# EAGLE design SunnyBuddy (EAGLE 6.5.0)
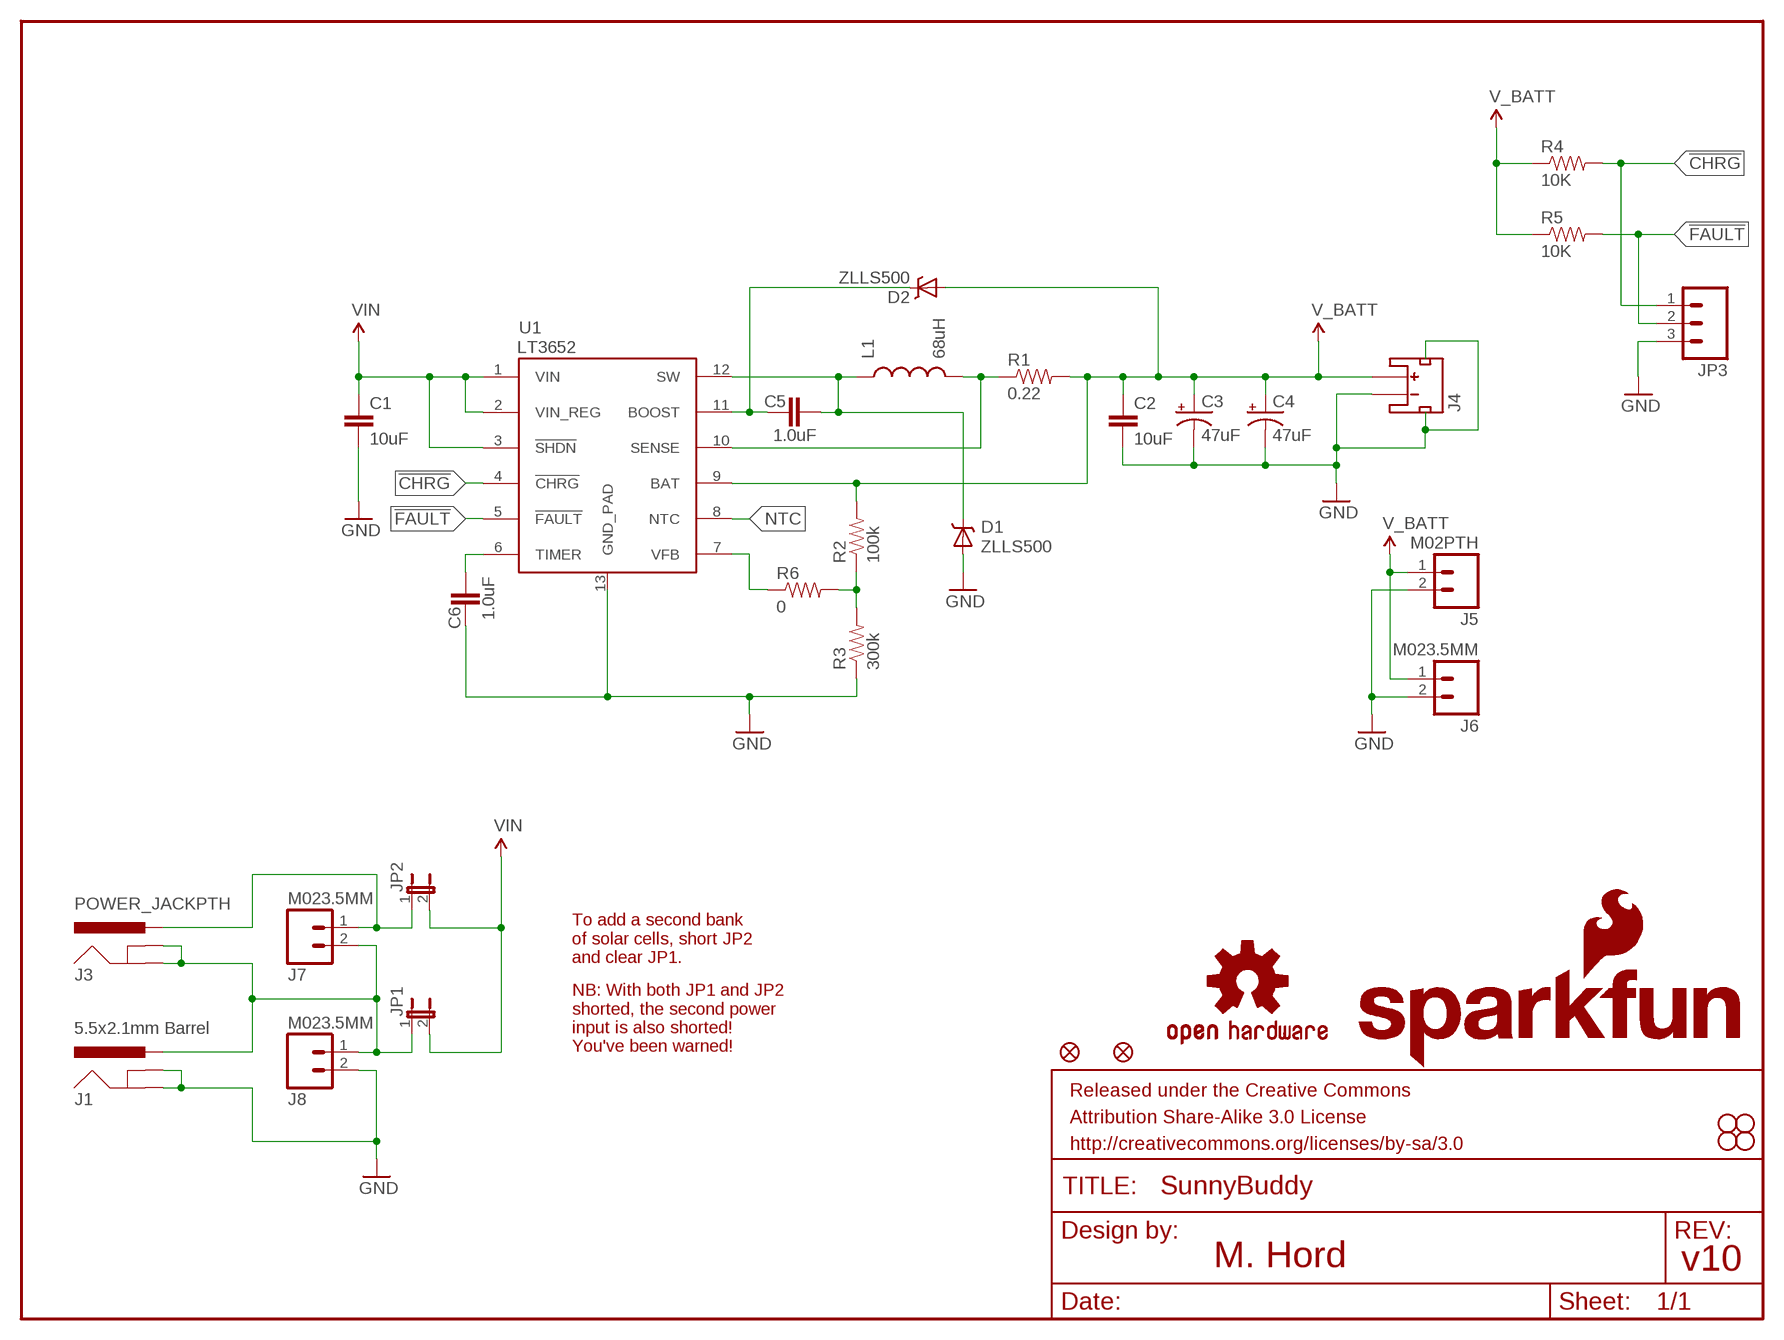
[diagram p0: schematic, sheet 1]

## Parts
C1  10uF  10UF50V20%(1210)  [1210]
C2  10uF  10UF-6.3V-20%(1206)  [1206]
C3  47uF  47UF-TANT  [EIA3528]
C4  47uF  47UF-TANT  [EIA3528]
C5  1.0uF  1.0UF-16V-10%(0603)  [0603-CAP]
C6  1.0uF  1.0UF-16V-10%(0603)  [0603-CAP]
D1  ZLLS500  ZLLS500ZLLS500  [SOT23]
D2  ZLLS500  ZLLS500ZLLS500  [SOT23]
FID1  FIDUCIAL1X2  [FIDUCIAL-1X2]
FID2  FIDUCIAL1X2  [FIDUCIAL-1X2]
FRAME1  FRAME-LETTER  [CREATIVE_COMMONS]
J1  5.5x2.1mm Barrel  POWER_JACKSMD  [POWER_JACK_SMD]
J3  POWER_JACKPTH  [POWER_JACK_PTH]
J4  JST_2MM_MALE  [JST-2-SMD]
J5  M02PTH  [1X02]
J6  M023.5MM  [SCREWTERMINAL-3.5MM-2]
J7  M023.5MM  [SCREWTERMINAL-3.5MM-2]
J8  M023.5MM  [SCREWTERMINAL-3.5MM-2]
JP1  JUMPER-2SMD-NC  [SJ_2S]
JP2  JUMPER-2SMD-NO  [SJ_2S-NO]
JP3  M03PTH  [1X03]
L1  68uH  INDUCTOR68UH-1A  [CR75]
LOGO1  SFE_LOGO_NAME_FLAME.2_INCH  [SFE_LOGO_NAME_FLAME_.2]
LOGO2  OSHW-LOGOM  [OSHW-LOGO-M]
R1  0.22  0.22OHM1/4W1%(0805)  [0805]
R2  100k  100KOHM1/10W1%(0603)  [0603-RES]
R3  300k  300KOHM-1/10W-1%(0603)  [0603-RES]
R4  10K  10KOHM1/10W1%(0603)0603  [0603-RES]
R5  10K  10KOHM1/10W1%(0603)0603  [0603-RES]
R6  0  0OHM1/10W5%(0603)  [0603]
STANDOFF1  STAND-OFF  [STAND-OFF]
STANDOFF2  STAND-OFF  [STAND-OFF]
STANDOFF3  STAND-OFF  [STAND-OFF]
STANDOFF4  STAND-OFF  [STAND-OFF]
U1  LT3652  [MSOP-12_GND]

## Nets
!CHRG: JP3.1 R4.2 U1.4(!CHRG)
!FAULT: JP3.2 R5.2 U1.5(!FAULT)
BOOST: C5.1 D2.3(C) U1.11(BOOST)
FB: R2.1 R3.2 R6.2
GND: C1.2 C2.2 C3.C(-) C4.C(-) C6.1 D1.1(A) J1.GND(GNDBREAK) J1.P$4(GND) J4.1(-) J4.NC1(PAD1) J4.NC2(PAD2) J5.2 J6.2 J8.2 JP3.3 R3.1 U1.13(GND_PAD)
N$3: R6.1 U1.7(VFB)
N$8: J1.VIN0(PWR) J3.GND J3.GNDBREAK J7.2 J8.1 JP1.1
NTC: U1.8(NTC)
SENSE: L1.P$2 R1.1 U1.10(SENSE)
SFSASDF: J3.PWR J7.1 JP2.1
SW: C5.2 D1.3(C) L1.P$1 U1.12(SW)
TIMER: C6.2 U1.6(TIMER)
V_BATT: C2.1 C3.A(+) C4.A(+) D2.1(A) J4.2(+) J5.1 J6.1 R1.2 R2.2 R4.1 R5.1 U1.9(BAT)
VIN: C1.1 JP1.2 JP2.2 U1.1(VIN) U1.2(VIN_REG) U1.3(!SHDN)

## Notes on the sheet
- To add a second bank
  of solar cells, short JP2
  and clear JP1.
- NB: With both JP1 and JP2
  shorted, the second power
  input is also shorted!
  You've been warned!
- M. Hord | v10

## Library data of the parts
C1 = SparkFun-Capacitors:10UF50V20%(1210): CAP-09824; PROD_ID: CAP-09824
C2 = SparkFun-Capacitors:10UF-6.3V-20%(1206): Ceramic; PROD_ID: CAP-10057
C3 C4 = SparkFun-Capacitors:47UF-TANT: 47uF Tantalum SMT; PROD_ID: CAP-08310
C5 C6 = SparkFun-Capacitors:1.0UF-16V-10%(0603): CAP-00868; PROD_ID: CAP-00868
D1 D2 = SparkFun-DiscreteSemi:ZLLS500: 700mA 40V SOT-23 Schottky; PROD_ID: DIO-08411
FID1 FID2 = SparkFun-Aesthetics:FIDUCIAL: Fiducial Alignment Points
FRAME1 = SparkFun-Aesthetics:FRAME-LETTER: Schematic Frame
J1 = SparkFun-Connectors:POWER_JACK: Power Jack This is the standard 5.5mm barrel jack for power. The PTH is the most common, proven, reliable, footprint. The Slot footprint only works if the mill layer is transmitted to the PCB fab house so be warned. Spark Fun Electronics SKU : PRT-00119 SMT: CONN-08106 Mating wall wart : TOL-00298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; PROD_ID: CONN-08106
J3 = SparkFun-Connectors:POWER_JACK: Power Jack This is the standard 5.5mm barrel jack for power. The PTH is the most common, proven, reliable, footprint. The Slot footprint only works if the mill layer is transmitted to the PCB fab house so be warned. Spark Fun Electronics SKU : PRT-00119 SMT: CONN-08106 Mating wall wart : TOL-00298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
J4 = SparkFun-Connectors:JST_2MM_MALE: Mates to single-cell LiPo batteries. CONN-08352; PROD_ID: CONN-08352
J5-J8 = SparkFun-Connectors:M02: Standard 2-pin 0.1" header. Use with
JP1 JP2 = SparkFun-Passives:JUMPER-2: Jumper
JP3 = SparkFun-Connectors:M03: Header 3 Standard 3-pin 0.1" header. Use with straight break away headers (SKU : PRT-00116), right angle break away headers (PRT-00553), swiss pins (PRT-00743), machine pins (PRT-00117), and female headers (PRT-00115). Molex polarized connector foot print use with SKU : PRT-08232 with associated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
L1 = SparkFun-Passives:INDUCTOR: Inductors; PROD_ID: NDUC-09739
LOGO1 = SparkFun-Aesthetics:SFE_LOGO_NAME_FLAME: SFE Logo, name and flame
LOGO2 = SparkFun-Aesthetics:OSHW-LOGO: Open Source Hardware Logo This logo indicates the piece of hardware it is found on incorporates a OSHW license and/or adheres to the definition of open source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
R1 = SparkFun-Resistors:0.22OHM1/4W1%(0805): RES-09883; PROD_ID: RES-09883
R2 = SparkFun-Resistors:100KOHM1/10W1%(0603): RES-07828; PROD_ID: RES-07828
R3 = SparkFun-Resistors:300KOHM-1/10W-1%(0603): RES-10809; PROD_ID: RES-10809
R4 R5 = SparkFun-Resistors:10KOHM1/10W1%(0603): RES-00824; PROD_ID: RES-00824
R6 = SparkFun-Resistors:0OHM1/10W5%(0603): RES-08609; PROD_ID: RES-08609
STANDOFF1-STANDOFF4 = SparkFun-Electromechanical:STAND-OFF: #4 Stand Off
U1 = SparkFun-PowerIC:LT3652: LT3652 MPPT Solar Charge Controller 5V-32V smart charger for batteries up to 14.4V

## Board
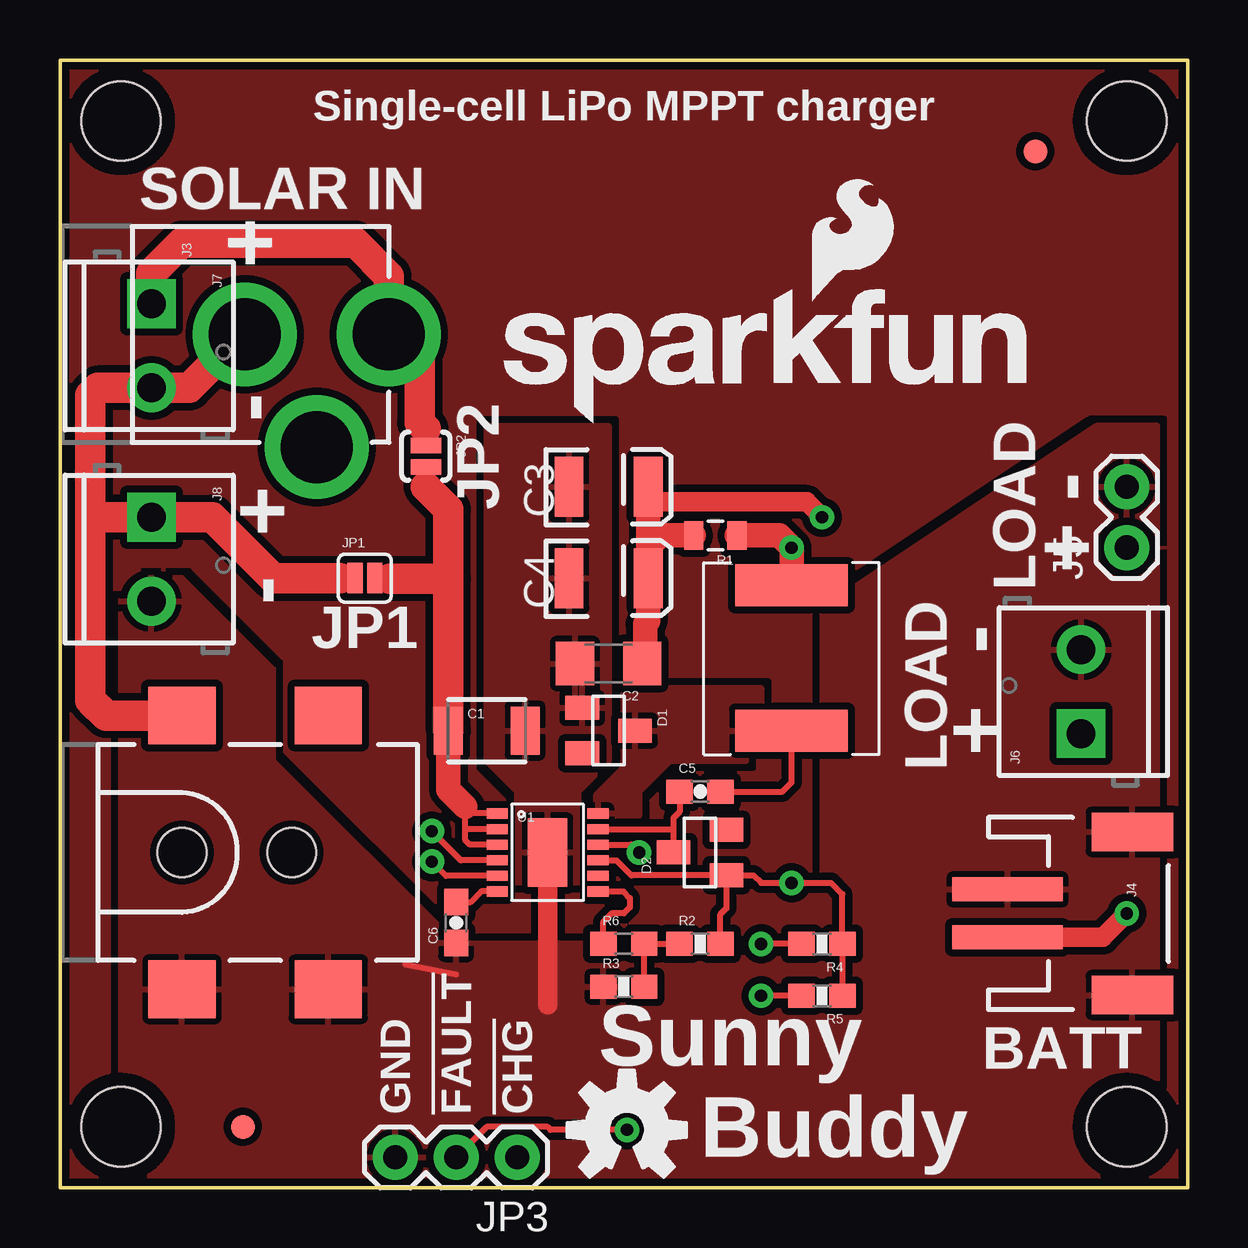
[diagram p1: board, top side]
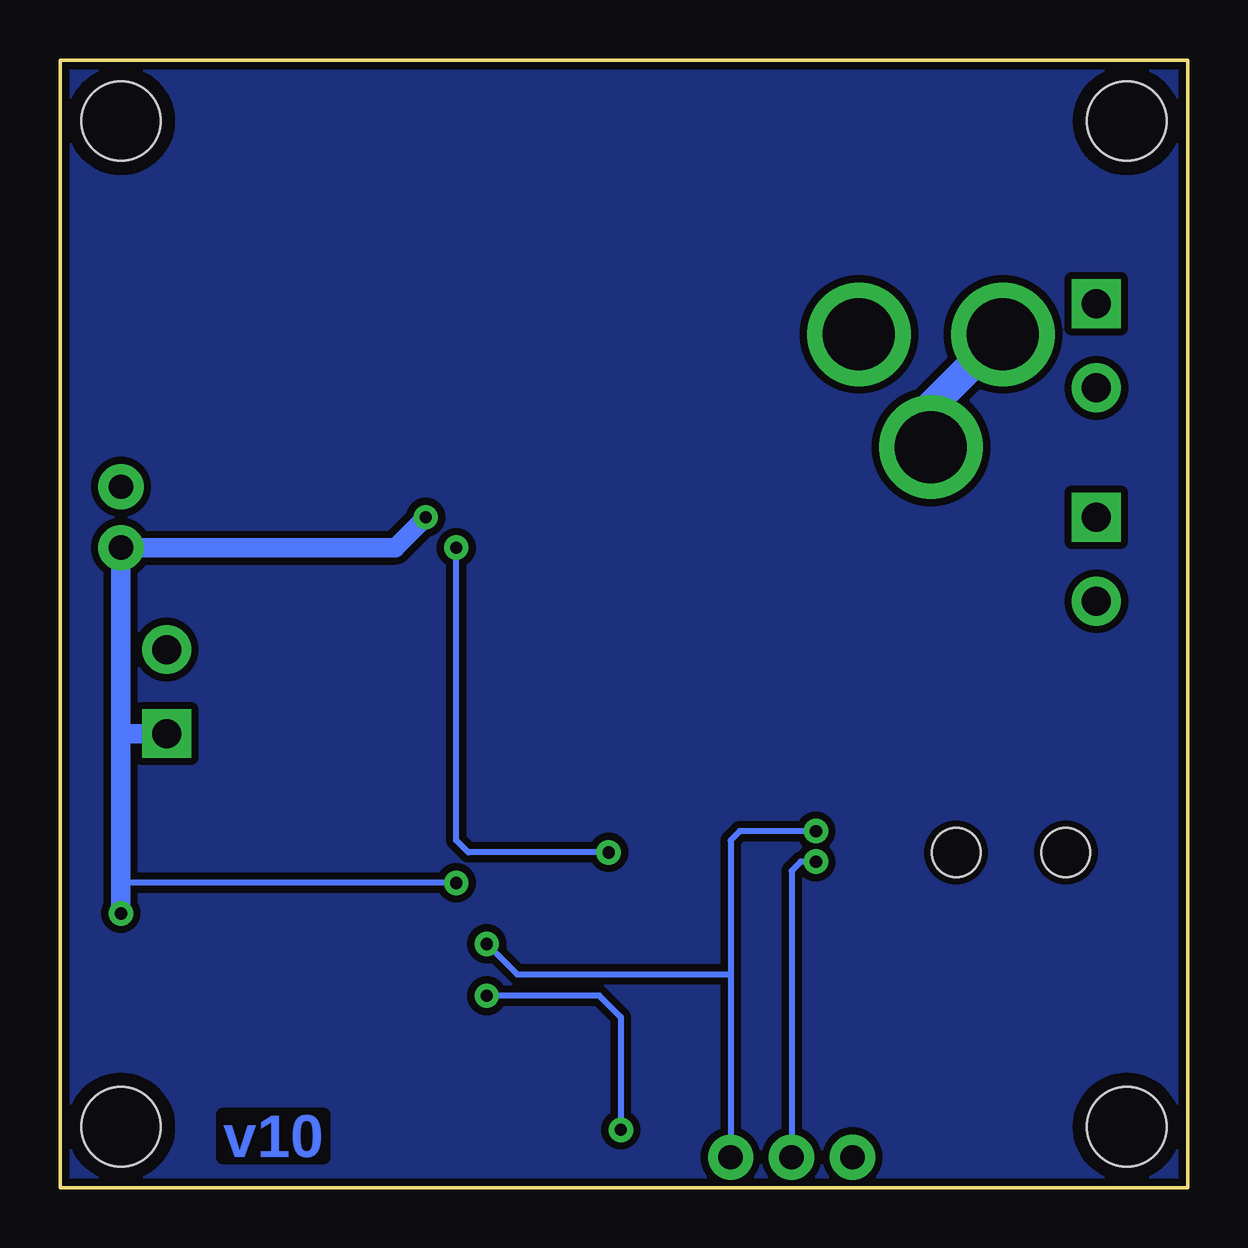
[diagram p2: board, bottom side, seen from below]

Size 46.99 x 46.99 mm. Coordinates in mm from the lower left corner, seen from the top.
Outline: 0,46.99 46.99,46.99 46.99,0 0,0 0,46.99
Copper layers (1*16): Top 0.035mm / dielectric 1.5mm / Bottom 0.035mm
Design rules "Sparkfun": minimum track width 8mil, minimum drill 20mil, track to track 8mil, track to pad 8mil, pad to pad 8mil, via to via 8mil, smd to smd 8mil, copper to edge 8mil, drill to drill 8mil, minimum pad ring 12mil, minimum via ring 10mil, stop-mask expansion 4mil, vias tented up to drill 20mil, thermal gap 10mil

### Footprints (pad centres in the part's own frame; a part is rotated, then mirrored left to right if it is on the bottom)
1210 = smd 1.2 x 2: 1 -1.6,0; 2 1.6,0
1206 = smd 1.6 x 1.8: 1 -1.4,0; 2 1.4,0
EIA3528 = smd 1.2 x 2.5: A 1.65,0; C -1.65,0
0603-CAP = smd 1.1 x 1: 1 -0.85,0; 2 0.85,0
SOT23 = smd 1 x 1.4: 1 -0.95,-1.1; 2 0.95,-1.1; 3 0,1.1
FIDUCIAL-1X2 = smd 1 x 1: 1 0,0
POWER_JACK_SMD = smd 2.8 x 2.4: GND 0,-5.7; P$4 6.1,-5.7; VIN0 0,5.7; VIN1 6.1,5.7 | hole 2.032: 0,0; 4.572,0
POWER_JACK_PTH = drill 2.997 pad 4.318: GND 0,7.7; GNDBREAK 4.7,10.7; PWR 0,13.7
JST-2-SMD = smd 1 x 4.6: 1 -1,-3.7; 2 1,-3.7 | smd 1.6 x 3.4: NC1 -3.4,1.5; NC2 3.4,1.5
1X02 = drill 1.016 pad 1.88: 1 0,0; 2 2.54,0
SCREWTERMINAL-3.5MM-2 = drill 1.2 pad 2.032 square: 1 0,0 | drill 1.2 pad 2.032: 2 3.5,0
SJ_2S = smd 0.635 x 1.27: 1 -0.412,0; 2 0.412,0
SJ_2S-NO = smd 0.635 x 1.27: 1 -0.45,0; 2 0.45,0
1X03 = drill 1.016 pad 1.88: 1 0,0; 2 2.54,0; 3 5.08,0
CR75 = smd 1.75 x 4.7: P$1 0,0; P$2 6.05,0
0805 = smd 0.8 x 1.2: 1 -0.9,0; 2 0.9,0
0603-RES = smd 1.1 x 1: 1 -0.85,0; 2 0.85,0
0603 = smd 1.1 x 1: 1 -0.85,0; 2 0.85,0
STAND-OFF = hole 3.302: 0,0
MSOP-12_GND = smd 0.889 x 0.42: 1 -2.1,1.625; 2 -2.1,0.975; 3 -2.1,0.325; 4 -2.1,-0.325; 5 -2.1,-0.975; 6 -2.1,-1.625; 7 2.1,-1.625; 8 2.1,-0.975; 9 2.1,-0.325; 10 2.1,0.325; 11 2.1,0.975; 12 2.1,1.625 | smd 1.651 x 2.845: 13 0,0

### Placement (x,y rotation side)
C1  17.78,19.05 0 top
C2  22.86,21.84 180 top
C3  22.86,29.21 0 top
C4  22.86,25.4 0 top
C5  26.67,16.51 0 top
C6  16.51,11.05 90 top
D1  22.86,19.05 270 top
D2  26.67,13.97 90 top
FID1  7.62,2.54 0 top
FID2  40.64,43.18 0 top
FRAME1  not placed on the board
J1  5.08,13.97 0 top
J3  0,35.56 270 top
J4  43.18,11.43 270 top
J5  44.45,26.67 90 top
J6  42.55,18.92 90 top
J7  3.81,36.83 270 top
J8  3.81,27.94 270 top
JP1  12.7,25.4 0 top
JP2  15.24,30.48 270 top
JP3  19.05,1.27 180 top
L1  30.48,19.05 90 top
LOGO1  17.78,31.75 0 top
LOGO2  23.62,2.41 0 top
R1  27.3,27.18 180 top
R2  26.67,10.16 0 top
R3  23.5,8.38 0 top
R4  31.75,10.16 180 top
R5  31.75,8 180 top
R6  23.5,10.16 0 top
STANDOFF1  2.54,2.54 0 top
STANDOFF2  2.54,44.45 0 top
STANDOFF3  44.45,44.45 0 top
STANDOFF4  44.45,2.54 0 top
U1  20.32,13.97 0 top

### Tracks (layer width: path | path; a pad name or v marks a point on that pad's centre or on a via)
!CHRG  (via drill 0.51)
  Top 0.254: U1.4 16.71,13.64 v15.49,14.86 | R4.2 v29.21,10.16
  Bottom 0.254: v15.49,14.86 18.67,14.86 19.05,14.48 19.05,8.89 | 19.05,8.89 JP3.1 | 19.05,8.89 27.94,8.89 v29.21,10.16
!FAULT  (via drill 0.51)
  Top 0.254: U1.5 16.09,12.99 v15.49,13.59 | v23.62,2.41 20.45,2.41 20.32,2.54 17.78,2.54 JP3.2 | R5.2 v29.21,8
  Bottom 0.254: v15.49,13.59 16.13,13.59 16.51,13.21 JP3.2 | v23.62,2.41 23.62,7.11 24.51,8 v29.21,8
BOOST
  Top 0.254: D2.3 25.57,14.86 | 25.57,14.86 25.57,15.41 25.82,15.66 C5.1 | U1.11 25.48,14.95 25.57,14.86
FB
  Top 0.254: R2.1 R6.2 R3.2
GND
  Top 0.254: 14.39,9.31 16.51,8.89
  Top 0.813: U1.13 20.32,7.62
  pour Top (isolate 0.305): 43.18,31.75 31.75,24.13 31.75,12.7 29.21,10.16 16.51,10.16 8.89,17.78 8.89,21.59 5.08,25.4 2.54,25.4 2.54,0 45.72,0 45.72,31.75
  pour Top (isolate 0.305): 22.86,31.75 22.86,17.78 21.59,16.51 21.59,12.7 19.05,12.7 19.05,16.51 17.78,17.78 17.78,31.75
N$1
  pour Top (isolate 0.305, rank 2, no thermals): 0,46.99 46.99,46.99 46.99,0 0,0
N$2
  pour Bottom (isolate 0.305, rank 2, no thermals): 0,46.99 46.99,46.99 46.99,0 0,0
N$3
  Top 0.254: U1.7 23.47,12.35 23.75,12.06 23.75,11.68 23.5,11.43 22.99,11.43 22.64,11.09 R6.1
N$8
  Top 0.254: J3.GND 7.62,35.56 | 11.68,25.4 JP1.1
  Top 1.27: 7.62,35.56 5.39,33.33 J7.2 1.58,33.33 1.27,33.02 1.27,27.94 | 1.27,27.94 1.27,20.32 1.92,19.67 J1.VIN0 | 11.68,25.4 8.89,25.4 6.35,27.94 J8.1 1.27,27.94
  Bottom 1.27: J3.GNDBREAK 10.7,32.56 J3.GND
SENSE  (via drill 0.51)
  Top 0.254: U1.10 23.8,14.29 v24.13,13.97
  Top 1.016: R1.1 29.97,27.18 v30.48,26.67 L1.P$2
  Bottom 0.254: v24.13,13.97 29.97,13.97 30.48,14.48 v30.48,26.67
SFSASDF
  Top 0.254: JP2.1 15.24,31.62
  Top 1.27: J7.1 3.81,38.1 5.08,39.37 12.32,39.37 13.7,37.99 J3.PWR 14.99,34.42 14.99,31.88 15.24,31.62
SW
  Top 0.254: C5.2 30.1,16.51 30.48,16.89 L1.P$1
  pour Top (isolate 0.305): 23.5,20.83 29.21,20.83 29.21,18.41 28.57,17.78 25.4,17.78 24.13,16.51 24.13,15.49 22.35,15.49 22.35,16.38 23.5,17.53
TIMER
  Top 0.254: U1.6 17.55,12.35 17.11,11.9 C6.2
V_BATT  (via drill 0.51)
  Top 0.254: U1.9 23.18,13.64 23.81,13.02 D2.1 | D2.1 28.89,13.02 29.21,12.7 v30.48,12.7 32.13,12.7 32.6,12.23 R4.1 R5.1 | 24.13,21.97 C2.1 | D2.1 27.77,11.64 27.52,11.39 R2.2
  Top 0.813: J4.2 43.45,10.43 v44.45,11.43 | C3.A 24.51,28.45 24.64,28.57 31.11,28.57 v31.75,27.94
  Top 1.016: 24.51,28.45 24.51,26.67 | 24.51,26.67 C4.A 24.51,23.62 24.38,23.5 24.38,21.97 C2.1 | R1.2 25.02,27.18 24.51,26.67
  Bottom 0.254: v30.48,12.7 44.45,12.7
  Bottom 0.813: v44.45,11.43 44.45,12.7 44.45,19.05 | 44.45,19.05 J5.1 33.02,26.67 v31.75,27.94 | J6.1 44.32,18.92 44.45,19.05
VIN
  Top 0.254: 13.73,25.39 13.72,25.4 JP1.2 | JP2.2 15.24,29.21 | U1.1 17.17,15.6 16.89,15.88 16.89,14.99 | U1.3 17.07,14.29 16.89,14.48 16.89,14.99 | U1.2 16.93,14.95 16.89,14.99
  Top 1.016: C1.1 16.18,16.59 16.89,15.88
  Top 1.27: C1.1 16.18,25.39 | 16.18,25.39 13.73,25.39 | 16.18,25.39 16.18,28.27 15.24,29.21

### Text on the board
Bottom: v10
tPlace: Single-cell LiPo MPPT charger | SOLAR IN | + | - | JP2 | - | + | + | - | LOAD | - | JP1 | + | LOAD | BATT | Sunny | GND | !FAULT | !CHG | Buddy
tDocu: M. Hord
